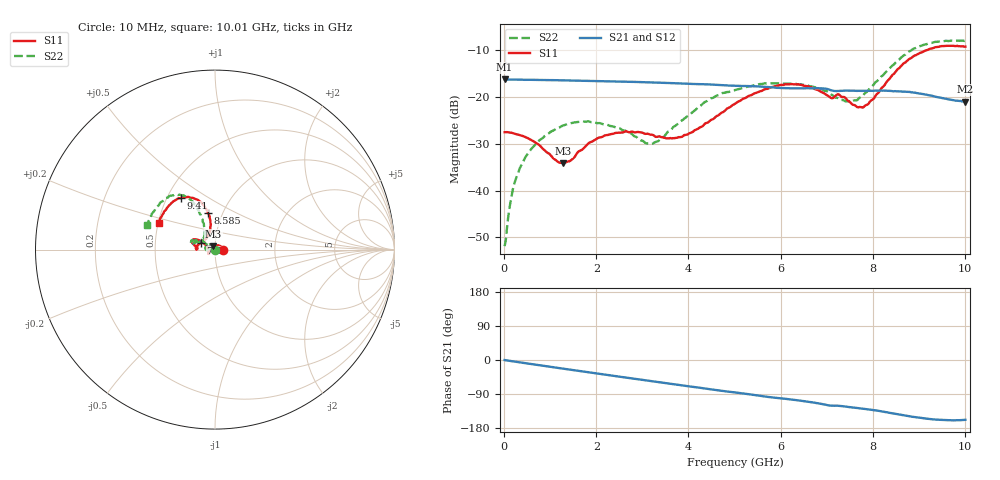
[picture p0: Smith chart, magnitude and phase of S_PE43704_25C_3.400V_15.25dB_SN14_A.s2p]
! Device ID: PE43704
! Dir: z:\PE43704\PE43704_Char_1_20130516\PE43704\AMB\3p400V\15p25dB
! Serial: 14
! Insertion: A
! Impedance: 50 ohm
! Temp: Amb
! VDD: 3.400V
! Attenuation Step: 15.25dB
! IDD: 1.139853e-01mA
#  Hz  S  RI  R  50
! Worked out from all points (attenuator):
!   401 points, 10 MHz to 10.01 GHz, reference 50 ohm
!   highest |S21| = -16.21 dB at 10 MHz (marker M1); lowest = -20.9 dB at 10.01 GHz (marker M2)
!   lowest |S11| = -34.1 dB at 1.285 GHz (marker M3), VSWR 1.04, Z = 49.1 + j1.73 ohm
!   |S11| at or under -10 dB: start of sweep to 9.149 GHz
!   |S22| runs from -51.9 to -7.9 dB; largest |S21 - S12| = 0.0013
!   S11 on the Smith chart (normalised r, x): 10 MHz: 1.09, +0.00; 7.51 GHz: 0.85, +0.06; 8.585 GHz: 0.85, +0.36; 9.41 GHz: 0.59, +0.38; 10.01 GHz: 0.50, +0.17
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1e7  0.0422 0.000245  0.1547 -0.000508  0.1548 -0.000479  -0.00249 0.000525
1.85e8  0.0407 0.00735  0.154 -0.00926  0.154 -0.00925  -0.00276 0.00977
4.1e8  0.0352 0.0153  0.1521 -0.0204  0.1522 -0.02  -0.00693 0.0191
7.35e8  0.0215 0.023  0.1489 -0.0351  0.1488 -0.0349  -0.0184 0.0279
1.285e9  -0.00888 0.0176  0.1395 -0.0589  0.1396 -0.0589  -0.0434 0.0244
1.685e9  -0.027 0.00385  0.1304 -0.0748  0.1303 -0.0748  -0.0539 0.0121
2.01e9  -0.0351 -0.00783  0.1214 -0.0866  0.1215 -0.0865  -0.0528 0.00239
2.435e9  -0.0366 -0.0197  0.1081 -0.1002  0.1081 -0.1002  -0.0469 -0.00334
3.11e9  -0.0337 -0.0228  0.0841 -0.1174  0.0842 -0.1173  -0.0314 0.00573
3.36e9  -0.0335 -0.0181  0.0744 -0.1221  0.0745 -0.122  -0.0316 0.0136
4.01e9  -0.0406 0.00489  0.0487 -0.1303  0.0488 -0.1302  -0.0537 0.0353
4.46e9  -0.0505 0.023  0.0308 -0.1333  0.031 -0.1335  -0.0786 0.0549
5.01e9  -0.073 0.0435  0.0102 -0.1322  0.0101 -0.1323  -0.1071 0.0522
5.96e9  -0.1209 0.0569  -0.0231 -0.1236  -0.0227 -0.1238  -0.1343 0.0399
6.685e9  -0.1226 0.0316  -0.0461 -0.1158  -0.0465 -0.1157  -0.1259 0.0328
7.51e9  -0.0801 0.0368  -0.0668 -0.0965  -0.0667 -0.0966  -0.0682 0.0581
7.835e9  -0.0458 0.0672  -0.0742 -0.0904  -0.0742 -0.0906  -0.0576 0.0949
8.36e9  -0.0255 0.1547  -0.0885 -0.0762  -0.0879 -0.0764  -0.0771 0.1859
8.585e9  -0.0399 0.2032  -0.0934 -0.0671  -0.0931 -0.0675  -0.1017 0.234
8.935e9  -0.0851 0.2685  -0.0976 -0.0537  -0.0974 -0.0527  -0.1635 0.2948
9.41e9  -0.1903 0.2872  -0.0926 -0.0382  -0.0926 -0.0379  -0.263 0.2905
1.001e10  -0.3142 0.1493  -0.0832 -0.0338  -0.084 -0.0339  -0.3768 0.136
